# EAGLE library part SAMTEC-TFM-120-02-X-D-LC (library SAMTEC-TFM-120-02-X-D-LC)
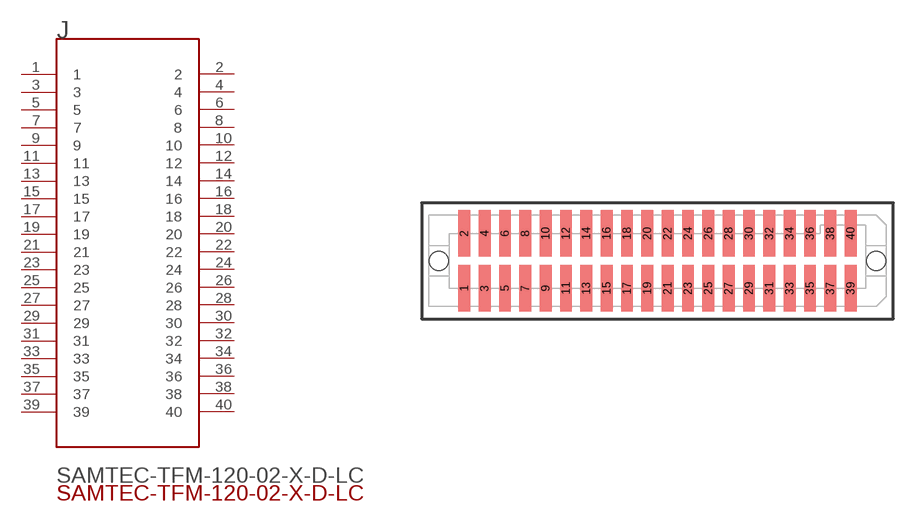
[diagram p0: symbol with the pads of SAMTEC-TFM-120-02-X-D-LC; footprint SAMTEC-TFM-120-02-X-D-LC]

Designator prefix J

## SAMTEC-TFM-120-02-X-D-LCJ (Description: HEADER, 1.27MM, SMT, 2X20POS; Series: TFM; Pitch Spacing: 1.27mm; No. of Rows: 2; N; Digi-Key_Part_Number: SAM10761-ND; Digi-Key_Purchase_URL: https://www.digikey.com/product-detail/en/samtec-inc/TFM-120-02-S-D-LC/SAM10761-ND/1952781?utm_source=snapeda&utm_medium=aggregator&utm_campaign=symbol; MF: Samtec; MP: TFM-120-02-S-D-LC; Package: None)  [SAMTEC-TFM-120-02-X-D-LC]
1  1  pas
2  2  pas
3  3  pas
4  4  pas
5  5  pas
6  6  pas
7  7  pas
8  8  pas
9  9  pas
10  10  pas
11  11  pas
12  12  pas
13  13  pas
14  14  pas
15  15  pas
16  16  pas
17  17  pas
18  18  pas
19  19  pas
20  20  pas
21  21  pas
22  22  pas
23  23  pas
24  24  pas
25  25  pas
26  26  pas
27  27  pas
28  28  pas
29  29  pas
30  30  pas
31  31  pas
32  32  pas
33  33  pas
34  34  pas
35  35  pas
36  36  pas
37  37  pas
38  38  pas
39  39  pas
40  40  pas

## Footprint SAMTEC-TFM-120-02-X-D-LC (pad centres in mm)
translated Allegro footprint
smd 0.74 x 2.92: 1 -12.065,-1.714; 2 -12.065,1.714; 3 -10.795,-1.714; 4 -10.795,1.714; 5 -9.525,-1.714; 6 -9.525,1.714; 7 -8.255,-1.714; 8 -8.255,1.714; 9 -6.985,-1.714; 10 -6.985,1.714; 11 -5.715,-1.714; 12 -5.715,1.714; 13 -4.445,-1.714; 14 -4.445,1.714; 15 -3.175,-1.714; 16 -3.175,1.714; 17 -1.905,-1.714; 18 -1.905,1.714; 19 -0.635,-1.714; 20 -0.635,1.714; 21 0.635,-1.714; 22 0.635,1.714; 23 1.905,-1.714; 24 1.905,1.714; 25 3.175,-1.714; 26 3.175,1.714; 27 4.445,-1.714; 28 4.445,1.714; 29 5.715,-1.714; 30 5.715,1.714; 31 6.985,-1.714; 32 6.985,1.714; 33 8.255,-1.714; 34 8.255,1.714; 35 9.525,-1.714; 36 9.525,1.714; 37 10.795,-1.714; 38 10.795,1.714; 39 12.065,-1.714; 40 12.065,1.714
hole 1.19 at 13.652,0
hole 1.19 at -13.652,0

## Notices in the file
This work is licensed under a Creative Commons Attribution-ShareAlike 4.0 International License (CC BY-SA) with Design Exception 1.0
